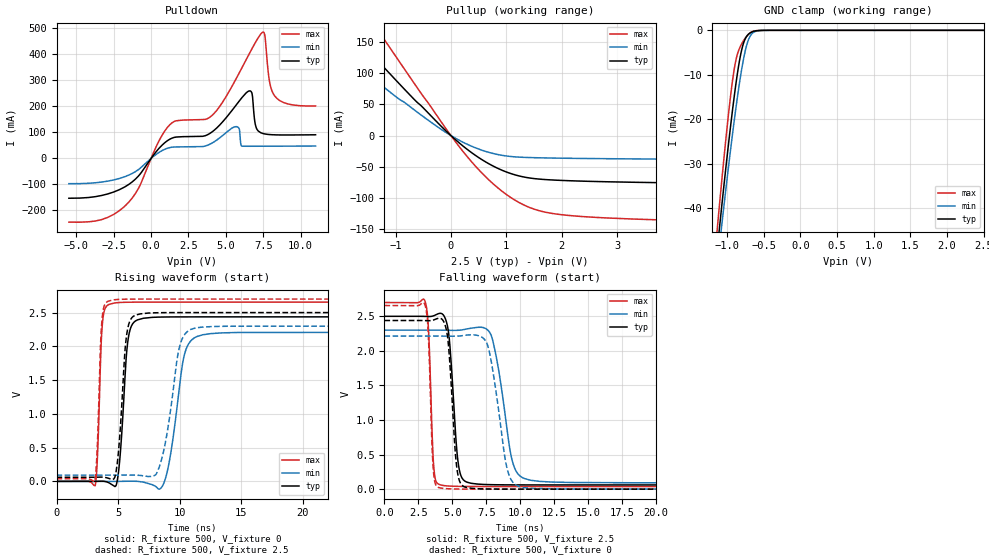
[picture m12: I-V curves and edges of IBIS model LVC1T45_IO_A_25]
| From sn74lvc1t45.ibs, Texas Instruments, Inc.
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[Model]   LVC1T45_IO_A_25
Model_type  I/O
Vinl=0.7
Vinh=1.7
Enable   Active-Low
Vref =   0
Rref =   2000
Cref =   15p
Vmeas =   1.25
| variable   typ   min   max
C_comp   7.12pF   6.25pF   8.15pF
| C_pullup   10.98pF   9.53pF   12.45pF
| C_pulldown   10.81pF   7.66pF   14.11pF
| C_tri-state   7.12pF   6.25pF   8.15pF
[Temperature Range]   40   100   -40
| Ambient temperature   25   85   -40
[Voltage range]   2.5   2.3   2.7
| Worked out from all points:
|   slope of the pulldown table from 0 to 0.375 V, typ, clamps not added: 13.2 ohm
|   slope of the pullup table from 0 to 0.375 V, typ, clamps not added: 13.6 ohm
|   GND clamp passes 1 mA (typ) near -0.71 V on its own axis
|   rising waveform, R_fixture 500, V_fixture 0: 20-80 % time 504ps typ, 960ps min, 286ps max; typ from 0 V to 2.44 V
|   falling waveform, R_fixture 500, V_fixture 2.5: 20-80 % time 493ps typ, 990ps min, 279ps max; typ from 2.5 V to 0.061 V
|   rising waveform, R_fixture 500, V_fixture 2.5: 20-80 % time 514ps typ, 1.04ns min, 289ps max; typ from 0.061 V to 2.5 V
|   falling waveform, R_fixture 500, V_fixture 0: 20-80 % time 468ps typ, 953ps min, 271ps max; typ from 2.44 V to 0 V
[GND Clamp]
| LVC1T45_IO_A_25
|   Voltage   I(typ)   I(min)   I(max)
-5.5V     -910.9mA   -836.3mA   -1.031A
-1.145V   -51.15mA   -54.65mA   -46.75mA
-1.11V    -45.51mA   -49.41mA   -40.47mA
-1.08V    -40.76mA   -44.98mA   -35.21mA
-1.065V   -38.41mA   -42.78mA   -32.63mA
-965mV    -23.43mA   -28.65mA   -16.64mA
-880mV    -12.18mA   -17.61mA   -6.789mA
-820mV    -5.939mA   -10.75mA   -3.68mA
-770mV    -2.643mA   -6.035mA   -2.191mA
-710mV    -920.7uA   -2.212mA   -923.3uA
-640mV    -245.9uA   -461.9uA   -195.8uA
2.5V      8.078pA    2.48nA     6.165pA
[Pulldown]
| LVC1T45_IO_A_25
|   Voltage   I(typ)   I(min)   I(max)
-5.5V     -153.1mA   -97.24mA   -245mA
-1.745V   -109.2mA   -70.16mA   -182.9mA
1.1V      68.14mA    38.92mA    119.4mA
4.065V    100.9mA    58.28mA    164mA
5.7V      205.5mA    121.8mA    307mA
6.545V    258.6mA    46.41mA    399.1mA
6.76V     245.7mA    46.42mA    422.2mA
7.015V    120.2mA    46.44mA    448.6mA
7.465V    95.59mA    46.5mA     484.5mA
7.93V     91.29mA    46.58mA    291.7mA
8.25V     90.27mA    46.64mA    240.6mA
11V       90.43mA    47.26mA    201.1mA
[Pullup]
| LVC1T45_IO_A_25
|   Voltage   I(typ)   I(min)   I(max)
-5.5V     488.5mA    380mA      648.9mA
-2.505V   233.8mA    173.3mA    321mA
-2.025V   188.1mA    137.6mA    260.7mA
-1.77V    163.6mA    118.6mA    228.1mA
-1.43V    130.8mA    93.6mA     184mA
-1.285V   116.8mA    83.09mA    165.1mA
-160mV    13.61mA    9.069mA    20.09mA
490mV     -34.67mA   -21.28mA   -53.66mA
1.11V     -61.84mA   -33.86mA   -101.2mA
1.715V    -70.74mA   -35.93mA   -123.3mA
3.895V    -75.85mA   -37.84mA   -135.8mA
11V       -81.86mA   -40.82mA   -147.4mA
[Ramp]
| LVC1T45_IO_A_25
| variable   typ   min   max
dV/dt_r   1.51/5.29E-10   1.39/1.02E-09   1.63/2.95E-10
dV/dt_f   1.49/5.06E-10   1.35/1.02E-09   1.63/2.88E-10
R_load = 500
[Rising Waveform]
| LVC1T45_IO_A_25
R_fixture =   500
C_fixture =   0
L_fixture =   0
V_fixture =   0
V_fixture_min = 0
V_fixture_max = 0
|   Time   V(typ)   V(min)   V(max)
0s        147.2pV    323.4pV    88.86pV
3.145ns   61.79uV    -7.514uV   -63.23mV
3.7ns     2.462mV    5.949uV    2.275V
4.3ns     -25.54mV   -38.69uV   2.624V
4.935ns   10.95mV    -56.44uV   2.647V
5.785ns   2.062V     1.909mV    2.653V
6.575ns   2.392V     375.2uV    2.654V
8.715ns   2.434V     -27.7mV    2.655V
11.41ns   2.436V     2.145V     2.655V
34.99ns   2.436V     2.208V     2.655V
[Falling Waveform]
| LVC1T45_IO_A_25
R_fixture =   500
C_fixture =   0
L_fixture =   0
V_fixture =   2.5
V_fixture_min = 2.3
V_fixture_max = 2.7
|   Time   V(typ)   V(min)   V(max)
0s        2.5V       2.3V       2.7V
3.01ns    2.499V     2.3V       2.708V
3.63ns    2.508V     2.3V       332.4mV
4.04ns    2.542V     2.3V       67.81mV
4.69ns    2.311V     2.298V     46.04mV
5.41ns    416.4mV    2.298V     40.64mV
6.07ns    101.9mV    2.317V     39.04mV
7.865ns   65.17mV    2.227V     38mV
10.33ns   61.54mV    152.7mV    37.85mV
34.99ns   61.03mV    92.13mV    37.77mV
[Rising Waveform]
| LVC1T45_IO_A_25
R_fixture =   500
C_fixture =   0
L_fixture =   0
V_fixture =   2.5
V_fixture_min = 2.3
V_fixture_max = 2.7
|   Time   V(typ)   V(min)   V(max)
0s        60.94mV    91.97mV    37.73mV
3.12ns    60.96mV    91.97mV    25.97mV
3.67ns    63.05mV    91.98mV    2.339V
4.22ns    45.42mV    91.96mV    2.67V
4.84ns    147.8mV    91.92mV    2.692V
5.67ns    2.133V     93.44mV    2.698V
6.395ns   2.461V     92.4mV     2.7V
8.345ns   2.498V     213.1mV    2.7V
10.93ns   2.5V       2.252V     2.7V
34.99ns   2.5V       2.3V       2.7V
[Falling Waveform]
| LVC1T45_IO_A_25
R_fixture =   500
C_fixture =   0
L_fixture =   0
V_fixture =   0
V_fixture_min = 0
V_fixture_max = 0
|   Time   V(typ)   V(min)   V(max)
0s        2.439V     2.214V     2.656V
2.995ns   2.438V     2.214V     2.662V
3.595ns   2.445V     2.215V     294.4mV
3.99ns    2.472V     2.214V     24.59mV
4.645ns   2.216V     2.213V     6.426mV
5.305ns   355.6mV    2.213V     2.41mV
5.905ns   32.45mV    2.225V     1.145mV
7.585ns   2.898mV    2.092V     249.4uV
9.885ns   410.3uV    41.58mV    112.5uV
34.99ns   75.23uV    139.9uV    38.24uV
